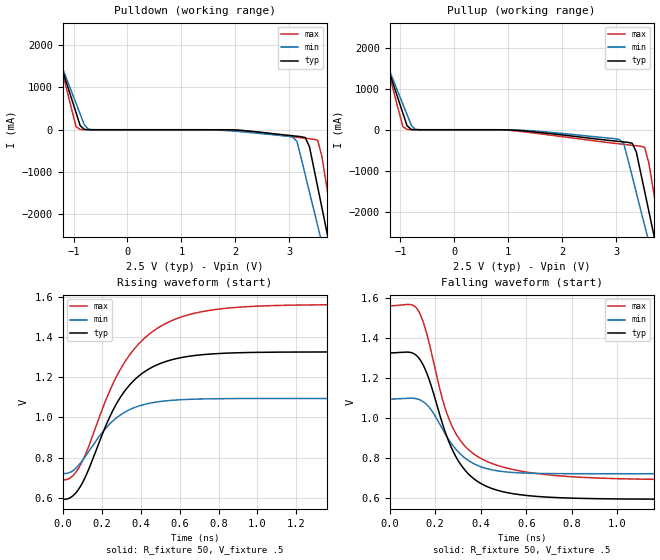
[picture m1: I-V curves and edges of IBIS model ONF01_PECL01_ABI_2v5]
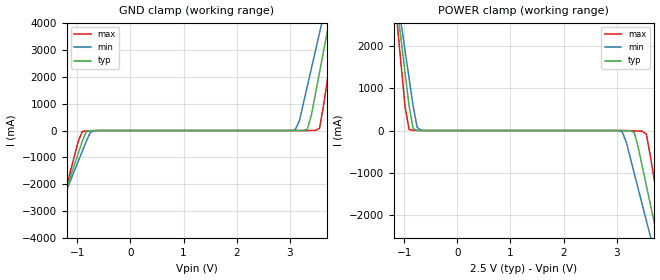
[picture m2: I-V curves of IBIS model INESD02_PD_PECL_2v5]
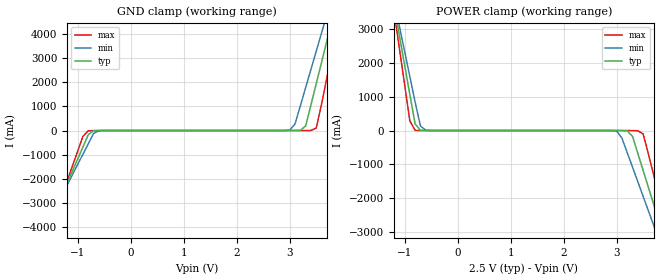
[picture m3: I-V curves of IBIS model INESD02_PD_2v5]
|   This file is an IBIS representation of the   |
|   Integrated Devices Technology, Inc.   |
|   ICS843004I   |
|   FEMTOCLOCKS CRYSTAL-TO-3.3V/2.5V LVPECL FREQUENCY SYNTHESIZER   |
[IBIS Ver]   4.1
[File name]   843004i.ibs
[File Rev]   1.0
[Date]   24 Dec 2008 | Last modified
|   24 Dec 2008 | Generated
[Source]   Originated at Integrated Devices Technology, Inc.
[Disclaimer]
IDT hereby grants the user of this IBIS model a non-exclusive,
nontransferable license to use this IBIS model under the following terms.
Before using this IBIS model, the user should read this license.
If the user does not accept these terms,  the IBIS model should be
returned to IDT within 30 days.
   The user is granted this license only to use the IBIS model and
is not granted rights to sell, load, rent, lease or license the IBIS
model in whole or in part, or in modified form to anyone other than
user. User may modify the IBIS model to suit its specific
applications but rights to derivative works and such modifications
shall belong to IDT.
   This IBIS model is provided on an "AS IS" basis and IDT makes
absolutely no warranty with respect to the information contained
herein. IDT DISCLAIMS AND CUSTOMER WAIVES ALL WARRANTIES, EXPRESS
OR IMPLIED, INCLUDING WARRANTIES OF MERCHANTABILITY OR FITNESS FOR
A PARTICULAR PURPOSE. The entire risk as to quality and performance
is with the Customer. ACCORDINGLY, IN NO EVENT SHALL THE COMPANY BE
LIABLE FOR ANY DAMAGES, WHETHER IN CONTRACT OR TORT,INCLUDING ANY
LOST PROFITS OR OTHER INCIDENTAL, CONSEQUENTIAL, EXEMPLARY, OR
PUNITIVE DAMAGES ARISING OUT OF THE USE OR APPLICATION OF THE IBIS
model provided in this package. Further, IDT reserves the right to
make changes without notice to any product herein to improve
reliability, function, or design. IDT does not convey any license
under patent rights or any other intellectual property rights,
including those of third parties.
   IDT is not obligated to provide maintenance or support
for the licensed IBIS model.
[Copyright]   Copyright 2004 byIntegrated Devices Technology, Inc.
[Component]   ICS843004I
[Manufacturer] Integrated Devices Technology, Inc.
[Package]
|TSSOP 24 Lead
|   typ   min   max
R_pkg   60.65m   52.4m   68.9m
L_pkg   1.989nH   1.431nH   2.547nH
C_pkg   0.314pF   0.254pF   0.374pF
[Pin]   signal_name   model_name   R_pin   L_pin   C_pin
1   nQ1   ONF01_PECL01_ABI   68.9m   2.547n   0.374p
2   Q1   ONF01_PECL01_ABI   65.6m   2.323n   0.350p
3   VCCO   POWER   62.3m   2.100n   0.326p
4   Q0   ONF01_PECL01_ABI   59.0m   1.877n   0.302p
5   nQ0   ONF01_PECL01_ABI   55.7m   1.654n   0.278p
6   MR   INESD02_PD_PECL   52.4m   1.431n   0.254p
7   nPLL_SEL   INESD02_PD   52.4m   1.431n   0.254p
8   NC   NC   55.7m   1.654n   0.278p
9   VCCA   POWER   59.0m   1.877n   0.302p
10  F_SEL0   INESD02_PD   62.3m   2.100n   0.326p
11  VCC   POWER   65.6m   2.323n   0.350p
12  F_SEL1   INESD02_PD   68.9m   2.547n   0.374p
13  XTAL_OUT   NC   68.9m   2.547n   0.374p
14  XTAL_IN   NC   65.6m   2.323n   0.350p
15  VEE   GND   62.3m   2.100n   0.326p
16  TEST_CLK   INESD02_PD_PECL   59.0m   1.877n   0.302p
17  nXTAL_SEL   INESD02_PD   55.7m   1.654n   0.278p
18  NC   NC   52.4m   1.431n   0.254p
19  VEE   GND   52.4m   1.431n   0.254p
20  nQ3   ONF01_PECL01_ABI   55.7m   1.654n   0.278p
21  Q3   ONF01_PECL01_ABI   59.0m   1.877n   0.302p
22  VCCO   POWER   62.3m   2.100n   0.326p
23  Q2   ONF01_PECL01_ABI   65.6m   2.323n   0.350p
24  nQ2   ONF01_PECL01_ABI   68.9m   2.547n   0.374p
[Diff Pin]  inv_pin  vdiff tdelay_typ tdelay_min  tdelay_max
2   1   NA   0   0   0
21   20   NA   0   0   0
23   24   NA   0   0   0
[Model Selector] ONF01_PECL01_ABI
ONF01_PECL01_ABI_2v5  Buffer selection for 2v5
ONF01_PECL01_ABI_3v3  Buffer selection for 3v3
[Model Selector] INESD02_PD_PECL
INESD02_PD_PECL_2v5  Buffer selection for 2v5
INESD02_PD_PECL_3v3  Buffer selection for 3v3
[Model Selector] INESD02_PD
INESD02_PD_2v5  Buffer selection for 2v5
INESD02_PD_3v3  Buffer selection for 3v3
| Models and submodels in the file (6): ONF01_PECL01_ABI_2v5 (Output_ECL), INESD02_PD_PECL_2v5 (Input), INESD02_PD_2v5 (Input), ONF01_PECL01_ABI_3v3 (Output_ECL), INESD02_PD_PECL_3v3 (Input), INESD02_PD_3v3 (Input)
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[Model] ONF01_PECL01_ABI_2v5
Model_type  Output_ECL
Polarity   Non-Inverting
Vmeas = .975
Rref = 50
Cref = 0
Vref = .5
|Variable  typ   min   max
C_comp   2p   1.5p   2.5p
[Voltage Range]   2.5   2.375   2.625
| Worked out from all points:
|   rising waveform, R_fixture 50, V_fixture .5: 20-80 % time 228ps typ, 199ps min, 276ps max; typ from 0.592 V to 1.33 V
|   falling waveform, R_fixture 50, V_fixture .5: 20-80 % time 153ps typ, 140ps min, 156ps max; typ from 1.33 V to 0.592 V
| Open source, no load
|  Voltage   I(typ)   I(min)   I(max)
[Pullup]
-2.5V     6.581A     5.758A     7.966A
-1.572V   2.868A     2.671A     3.219A
-1.418V   2.25A      2.158A     2.429A
-953.6mV  402.1mA    621.9mA    72.14mA
-876.3mV  95.6mA     366.6mA    5.897mA
-721.6mV  951.4uA    9.59mA     751.4uA
3.067V    -287.8mA   -237.7mA   -346mA
3.299V    -330.4mA   -1.134A    -380.1mA
3.531V    -1.506A    -2.34A     -427.9mA
3.686V    -2.47A     -3.144A    -1.427A
3.84V     -3.434A    -3.947A    -2.655A
5V        -10.66A    -9.976A    -11.86A
[Pulldown]
-2.5V     6.581A     5.758A     7.966A
-1.495V   2.559A     2.415A     2.824A
-1.418V   2.25A      2.158A     2.429A
-953.6mV  402.1mA    621.9mA    72.14mA
-876.3mV  95.6mA     366.6mA    5.897mA
-721.6mV  951.4uA    9.59mA     751.4uA
3.067V    -142.9mA   -171.4mA   -166.7mA
3.299V    -185mA     -1.067A    -201.5mA
3.531V    -1.361A    -2.272A    -250mA
3.686V    -2.324A    -3.076A    -1.249A
3.84V     -3.288A    -3.879A    -2.478A
5V        -10.51A    -9.904A    -11.69A
[Ramp]
|   typ   min   max
dV/dt_r   0.586/0.368n   0.299/0.313n   0.698/0.446n
dV/dt_f   0.590/0.258n   0.302/0.226n   0.703/0.290n
R_load =   50.0000
[Rising Waveform]
R_fixture = 50
V_fixture = .5   | VCC_typ - 2V
V_fixture_max = 0.625   | VCC_max - 2V
V_fixture_min = 0.375   | VCC_min - 2V
C_fixture = 0.0p
| Time   typ   min   max
0s        592.5mV    720.8mV    689.3mV
46.2ps    605.5mV    731.1mV    704.8mV
92.4ps    659.4mV    774.5mV    766.4mV
241.5ps   1.003V     967.6mV    1.133V
323.4ps   1.138V     1.029V     1.283V
426.3ps   1.231V     1.066V     1.4V
552.3ps   1.285V     1.084V     1.478V
711.9ps   1.312V     1.092V     1.525V
940.8ps   1.323V     1.094V     1.551V
1.999ns   1.326V     1.094V     1.562V
[Falling Waveform]
R_fixture = 50
V_fixture = .5   | VCC_typ - 2V
V_fixture_max = 0.625   | VCC_max - 2V
V_fixture_min = 0.375   | VCC_min - 2V
C_fixture = 0.0p
| Time   typ   min   max
0s        1.326V     1.094V     1.562V
92.4ps    1.328V     1.099V     1.568V
123.9ps   1.306V     1.095V     1.541V
168ps     1.209V     1.061V     1.4V
231ps     973.8mV    945.4mV    1.097V
277.2ps   835.9mV    862.7mV    951mV
348.6ps   716.5mV    784.8mV    838.7mV
447.3ps   647.2mV    740.6mV    773mV
865.2ps   596.5mV    720.8mV    701.4mV
1.999ns   592.4mV    720.7mV    689.3mV
[Model] INESD02_PD_PECL_2v5
Model_type   Input
Polarity   Non-Inverting
Vinl = 0.8V
Vinh = 2.0V
|   typ   min   max
C_comp   2pF   1.5pF   2.5pF
|   typ   min   max
[Voltage range]  2.5V   2.375V   2.625V
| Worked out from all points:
|   GND clamp passes 1 mA (typ) near -0.59 V on its own axis
|   POWER clamp passes 1 mA (typ) near -0.69 V on its own axis
[GND_clamp]
|Voltage   I(typ)   I(min)   I(max)
-2.5V     -9.799A    -8.591A    -11.84A
-1.591V   -4.431A    -4.121A    -4.98A
-1.439V   -3.536A    -3.377A    -3.837A
-909.1mV  -407.1mA   -774.3mA   -35.24mA
-833.3mV  -48.47mA   -403.4mA   -14.47mA
-681.8mV  -2.863mA   -7.067mA   -5.73mA
3.106V    167.2uA    32.81mA    49.66uA
3.333V    47.81mA    1.661A     649.6uA
3.561V    2.15A      3.618A     75.79mA
3.712V    3.718A     4.923A     1.92A
3.864V    5.287A     6.229A     3.927A
5V        17.07A     16.03A     18.99A
[POWER_clamp]
|Voltage   I(typ)   I(min)   I(max)
-2.5V     17.07A     14.96A     20.65A
-1.136V   2.934A     3.193A     2.572A
-1.061V   2.15A      2.541A     1.569A
-909.1mV  582.4mA    1.237A     24.21mA
-833.3mV  47.81mA    585.7mA    3.595mA
-681.8mV  586.4uA    6.896mA    416.8uA
3.106V    -1.127mA   -30.71mA   -286.5uA
3.333V    -48.47mA   -1.016A    -7.036mA
3.485V    -853.6mA   -1.759A    -17.14mA
3.712V    -2.194A    -2.874A    -1.179A
3.939V    -3.536A    -3.991A    -2.894A
5V        -9.799A    -9.206A    -10.89A
[Model] INESD02_PD_2v5
Model_type   Input
Polarity   Non-Inverting
Vinl = 1.4V
Vinh = 1.85V
|   typ   min   max
C_comp   2pF   1.5pF   2.5pF
|   typ   min   max
[Voltage range]  2.5V   2.375V   2.625V
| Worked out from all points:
|   GND clamp passes 1 mA (typ) near -0.55 V on its own axis
|   POWER clamp passes 1 mA (typ) near -0.60 V on its own axis
[GND_clamp]
|Voltage I(typ)   I(min)   I(max)
-2.5V     -8.775A    -7.892A    -10.18A
-1.6V     -4.218A    -4.001A    -4.586A
-900mV    -678.5mA   -979.3mA   -237.6mA
-800mV    -173.9mA   -548.7mA   -10.83mA
-600mV    -1.629mA   -8.74mA    -911.1uA
3V        133.3uA    17.16mA    56.6uA
3.1V      660.9uA    273.5mA    60.87uA
3.3V      191.6mA    1.785A     327.9uA
3.5V      1.949A     3.298A     103.6mA
3.7V      3.723A     4.812A     2.189A
3.9V      5.498A     6.327A     4.369A
5V        15.27A     14.67A     16.38A
[POWER_clamp]
|Voltage   I(typ)   I(min)   I(max)
-2.5V     15.27A     13.72A     17.74A
-1.2V     3.723A     3.866A     3.551A
-1.1V     2.836A     3.109A     2.461A
-900mV    1.063A     1.596A     283.3mA
-800mV    191.6mA    840.1mA    6.189mA
-600mV    660.9uA    8.845mA    114.2uA
3V        -338.1uA   -16.36mA   -12.68uA
3.4V      -678.5mA   -1.518A    -7.183mA
3.5V      -1.183A    -1.95A     -99.52mA
3.7V      -2.195A    -2.813A    -1.324A
4V        -3.712A    -4.109A    -3.188A
5V        -8.775A    -8.432A    -9.404A
